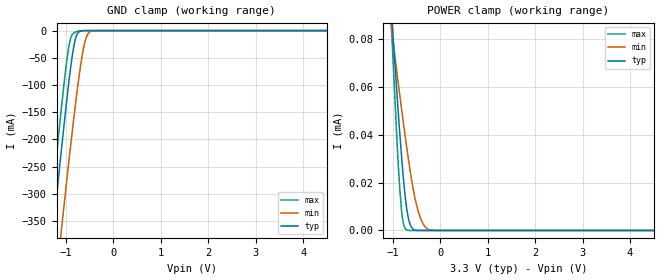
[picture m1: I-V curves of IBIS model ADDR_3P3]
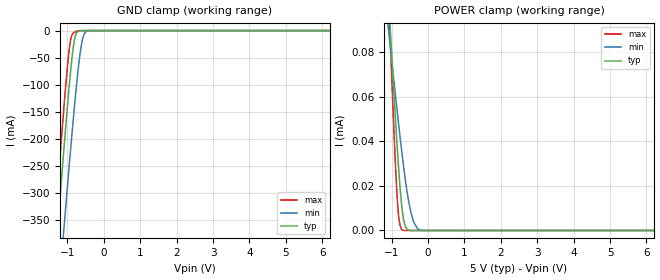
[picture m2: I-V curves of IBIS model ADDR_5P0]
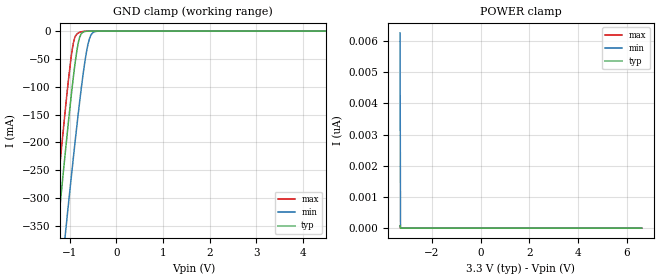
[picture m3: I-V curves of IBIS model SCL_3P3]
| Texas Instruments Incorporated
| 11-to-14 Bit Digital Temperature Sensor with 2-Wire Interface
| Marketing part#   Voltage Range   Package-type   #pins/pkg drawing
| LM73CIMK   2.7V - 5.5V   SOT   6-pin CIMK
[IBIS Ver]   4.1
[File name]   lm73.ibs
[File Rev]   1.0
[Date]   12/02/2013
[Source]   Model built from spectre simulations at:
   Texas Instruments Incorporated.
   Analog-eLab, HPA
   12500 TI Blvd
   Dallas, TX -75243
   For Support e-mail: elab_ibis@list.ti.com
[Notes]   Revision History
   Rev 1.0: 12/02/2013
   - ccomp values are based on PVT settings:
   MIN: Low Voltage, High Temperature, Weak Process
   TYP: Nominal Voltage, Nominal Temperature, Nominal Process
   MAX: High Voltage, Low Temperature, Fast Process
   - C_comp although listed in numerical order of value are obtained from varying PVT conditions.
   For PVT conditions for each specific value, refer to the buffer description under respective [Model].
   IBIS model user is responsible for using appropriate C_comp to simulate for Signal Integrity.
[Disclaimer]  This model is designed as an aid for customers of Texas Instruments
 TI and its licensors and suppliers make no warranties, either expressed
 or implied, with respect to this  model, including the warranties of
 merchantability or fitness for a particular purpose.
 The model is provided solely on an "as is" basis. The entire risk as to
 its quality and performance is with the customer.
[Copyright] (C)Copyright 2013 Texas Instruments Incorporated.
   All rights reserved.
[Component]   LM73CIMK
[Manufacturer]  Texas Instruments Incorporated
[Package]   |6-pin SOT package
|   typ   min   max
R_pkg   0.0901   0.0864   0.0947
L_pkg   1.7958n   1.7001n   1.9475n
C_pkg   0.3093p   0.2684p   0.4851p
[Pin]   signal_name   model_name   R_pin   L_pin   C_pin
1   ADDR   ADDR   0.08989  1.70368n  0.26894p
2   GND   GND   0.09071  1.83871n  0.48514p
3   VDD   POWER   0.08957  1.70014n  0.26841p
4   SMBCLK   SCL   0.08638  1.85659n  0.27368p
5   ALERTB   ALERT   0.08944  1.72798n  0.28039p
6   SMBDAT   SDA   0.09466  1.94746n  0.27907p
[Model Selector] ADDR
ADDR_3P3   ADDR 3.3V INPUT
ADDR_5P0   ADDR 5V INPUT
[Model Selector] SCL
SCL_3P3   SCL 3.3V INPUT
SCL_5P0   SCL 5V INPUT
[Model Selector] SDA
SDA_3P3   SDA 3.3V OPEN-DRAIN I/O
SDA_5P0   SDA 5V OPEN-DRAIN I/O
[Model Selector] ALERT
ALERT_3P3   ALERT 3.3V OPEN-DRAIN OUTPUT
ALERT_5P0   ALERT 5V OPEN-DRAIN OUTPUT
| Models and submodels in the file (8): ADDR_3P3 (Input), ADDR_5P0 (Input), SCL_3P3 (Input), SCL_5P0 (Input), ALERT_3P3 (Open_drain), ALERT_5P0 (Open_drain), SDA_3P3 (I/O_open_drain), SDA_5P0 (I/O_open_drain)
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|   (nom PVT)   (slow PVT)   (fast PVT)
|   Model ADDR_3P3
[Model]   ADDR_3P3
Model_type   Input
Vinl = 0.99
Vinh = 2.31
|   typ   min   max
|   (nom PVT)   (fast PVT)   (slow PVT)
C_comp   0.4295pF   0.3981pF   0.4645pF
[Model spec]
|subparameter
Vinl   0.99   0.81   1.08
Vinh   2.31   1.89   2.52
[Voltage Range]   3.3   2.7   3.6
[Temperature Range]   27   150   -40
[Power Clamp Reference]   3.3   2.7   3.6
[GND Clamp Reference]   0   0   0
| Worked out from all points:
|   GND clamp passes 1 mA (typ) near -0.69 V on its own axis
[GND Clamp]
|   Voltage   I(typ)   I(min)   I(max)
-3.3V     -2.187A    -2.242A    -2.165A
-1.379V   -461.8mA   -601mA     -389.4mA
-1.29V    -383.9mA   -526.1mA   -309.5mA
-1.112V   -231.4mA   -378.5mA   -154.7mA
-993.3mV  -134.9mA   -282.6mA   -61.84mA
-933.9mV  -90.16mA   -235.8mA   -26.3mA
-874.5mV  -50.28mA   -190.1mA   -8.277mA
-795.3mV  -13.32mA   -131.8mA   -2.478mA
-617.1mV  -161.4uA   -26.72mA   -53.95uA
-547.8mV  -25.92uA   -7.583mA   -6.702uA
-448.8mV  -1.464uA   -700.5uA   -202.6nA
6.6V      0A         0A         0A
[POWER Clamp]
|   Voltage   I(typ)   I(min)   I(max)
-3.3V     737uA      433.3uA    1.029mA
-1.023V   88.91uA    83.11uA    82.28uA
-1.013V   85.94uA    81.52uA    77.99uA
-904.2mV  54.16uA    64.19uA    33.68uA
-854.7mV  40.56uA    56.48uA    17.22uA
-785.4mV  23.33uA    45.93uA    3.627uA
-706.2mV  8.744uA    34.41uA    219.8nA
-617.1mV  1.686uA    22.61uA    0A
-498.3mV  28.47nA    10.35uA    0A
-389.4mV  0A         3.753uA    0A
-250.8mV  0A         368.7nA    0A
6.6V      0A         0A         0A
|   Model ADDR_5P0
[Model]   ADDR_5P0
Model_type   Input
Vinl = 1.5
Vinh = 3.5
|   typ   min   max
|   (nom PVT)   (fast PVT)   (slow PVT)
C_comp   0.4295pF   0.3981pF   0.4645pF
[Model spec]
|subparameter
Vinl   1.5   1.35   1.65
Vinh   3.5   3.15   3.85
[Voltage Range]   5   4.5   5.5
[Temperature Range]   27   150   -40
[Power Clamp Reference]   5   4.5   5.5
[GND Clamp Reference]   0   0   0
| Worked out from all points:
|   GND clamp passes 1 mA (typ) near -0.69 V on its own axis
[GND Clamp]
|   Voltage   I(typ)   I(min)   I(max)
-5V       -3.717A    -3.696A    -3.741A
-1.355V   -440.4mA   -580.4mA   -367.4mA
-1.25V    -348.9mA   -492.5mA   -273.8mA
-1.1V     -221.3mA   -368.7mA   -144.6mA
-995mV    -136.2mA   -283.9mA   -63.02mA
-920mV    -80.27mA   -225mA     -20.27mA
-830mV    -26.35mA   -156.9mA   -4.054mA
-755mV    -5.09mA    -103.9mA   -1.322mA
-665mV    -538.9uA   -48.98mA   -194.9uA
-590mV    -80.13uA   -17.28mA   -24.68uA
-425mV    -679.3nA   -381.2uA   -60.97nA
10V       0A         0A         0A
[POWER Clamp]
|   Voltage   I(typ)   I(min)   I(max)
-5V       1.038mA    614.9uA    1.425mA
-1.115V   113uA      94.44uA    118.8uA
-1.04V    90.98uA    82.76uA    86.6uA
-920mV    56.84uA    64.34uA    38.42uA
-830mV    33.18uA    50.89uA    10.64uA
-770mV    19.49uA    42.2uA     2.305uA
-680mV    5.665uA    29.86uA    50.99nA
-590mV    854.6nA    18.9uA     0A
-455mV    0A         7.119uA    0A
-290mV    0A         834.9nA    0A
-200mV    0A         95.93nA    0A
10V       0A         0A         0A
|   Model SCL_3P3
[Model]   SCL_3P3
Model_type   Input
Vinl = 0.99
Vinh = 2.31
|   typ   min   max
|   (nom PVT)   (fast PVT)   (slow PVT)
C_comp   0.4295pF   0.3981pF   0.4645pF
[Model spec]
|subparameter
Vinl   0.99   0.81   1.08
Vinh   2.31   1.89   2.52
[Voltage Range]   3.3   2.7   3.6
[Temperature Range]   27   150   -40
[Power Clamp Reference]   3.3   2.7   3.6
[GND Clamp Reference]   0   0   0
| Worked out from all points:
|   GND clamp passes 1 mA (typ) near -0.69 V on its own axis
[GND Clamp]
|   Voltage   I(typ)   I(min)   I(max)
-3.3V     -2.187A    -2.242A    -2.165A
-1.379V   -461.9mA   -601mA     -389.4mA
-1.29V    -383.9mA   -526.2mA   -309.6mA
-1.201V   -306.9mA   -452mA     -231mA
-1.112V   -231.4mA   -378.6mA   -154.8mA
-1.053V   -182.4mA   -330.3mA   -106.4mA
-924mV    -83.17mA   -228.1mA   -22.01mA
-795.3mV  -13.4mA    -131.9mA   -2.481mA
-617.1mV  -161.6uA   -26.78mA   -53.95uA
-547.8mV  -25.87uA   -7.625mA   -6.699uA
-448.8mV  -1.46uA    -706.4uA   -200.3nA
6.6V      0A         0A         0A
[POWER Clamp]
|   Voltage   I(typ)   I(min)   I(max)
-3.3V     74.18pA    6.26nA     75.92pA
-3.28V    0A         0A         0A
-3.27V    0A         0A         0A
6.6V      0A         0A         0A
